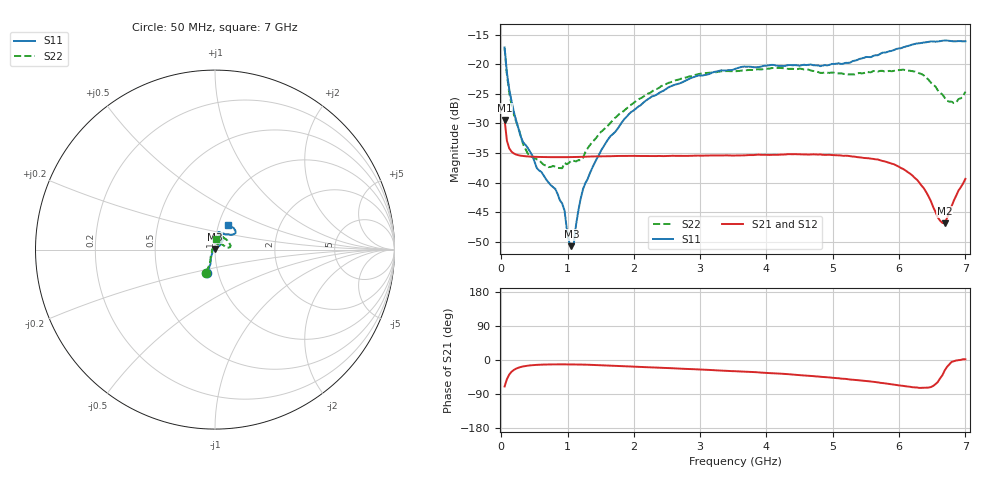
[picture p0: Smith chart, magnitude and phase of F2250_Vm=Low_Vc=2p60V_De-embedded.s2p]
! Integrated Device Technology
! Corporate Headquarters
! 6024 Silver Creek Valley Road
! San Jose, CA 95138  USA
! Phone:  1-408-284-8200
! Toll Free:  1-800-223-1366
! Webpage:  http://www.idt.com/
! Timing and RF Division
! 515 Groton Road, Suite 102
! Westford, MA 01886-6024
! Device:  F2250
! Description: Voltage Variable RF Attenuator
! Frequency:  50.0 -  6000.00 MHz
! Package:  3x3 mm Thin QFN Plastic Package: 16 pin
! Ports:  2 RF, 3 DC
!  Pin  1  = GND
!  Pin  2  = NC
!  Pin  3  = RF1  = Port 1
!  Pin  4  = NC
!  Pin  5  = GND
!  Pin  6  = GND
!  Pin  7  = GND
!  Pin  8  = GND
!  Pin  9  = NC
!  Pin 10  = RF2  = Port 2
!  Pin 11  = NC
!  Pin 12  = GND
!  Pin 13  = GND
!  Pin 14  = VCNTRL
!  Pin 15  = VDD
!  Pin 16  = VMODE
! Vcntrl:  2.600 Volts
! Vmode:  +0.000 Volts
! Vdd:  +3.30  Volts
! Current:  1.176 mA
! Data:  The device was measured on a the F2250 evaluation board which has
!  individual transmission lines to the RF pins.  Data was collected
!  using a calibrated network analyzer.  The evaluation board was
!  de-embedded using a TRL calibration technique.
!  The reference plane is the edge of the package pin.
! Misc:  SN 10
!  Action Tracker AT0258
! Date Measured:  2014-11-26
! Date:  2015-10-15  MJV
! Note:
!  Integrated Device Technology supplies this data as a sample of measured
!  data at the package pin for this product.  Your particular data for this
!  product may vary.
!  Data was taken at 25 degrees C.
!  Integrated Device Technology reserves the right to change this data at anytime.
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# GHz S dB R 50
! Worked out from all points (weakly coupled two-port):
!   201 points, 50 MHz to 7 GHz, reference 50 ohm
!   highest |S21| = -29.41 dB at 50 MHz (marker M1); lowest = -46.8 dB at 6.687 GHz (marker M2)
!   lowest |S11| = -50.7 dB at 1.058 GHz (marker M3), VSWR 1.01, Z = 49.8 + j0.243 ohm
!   |S11| at or under -10 dB: start of sweep to end of sweep
!   |S22| runs from -37.5 to -17.3 dB; largest |S21 - S12| = 6.2e-05
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0.05  -17.18 -108.6  -29.41 -69.8  -29.41 -69.8  -17.28 -111.0
0.08475  -21.45 -107.5  -32.92 -50.4  -32.92 -50.4  -21.74 -110.2
0.15425  -26.23 -116.6  -34.76 -31.1  -34.75 -31.2  -26.81 -122.5
0.29325  -32.21 -127.8  -35.43 -18.5  -35.43 -18.5  -32.09 -137.4
0.3975  -34.09 -141.7  -35.56 -15.0  -35.56 -15.0  -35.05 -160.5
0.91875  -43.51 157.9  -35.69 -11.5  -35.69 -11.5  -37.54 133.5
0.9535  -44.66 170.2  -35.68 -11.5  -35.68 -11.5  -36.65 131.0
1.023  -49.98 143.9  -35.67 -11.6  -35.67 -11.6  -36.63 115.9
1.05775  -50.70 123.4  -35.67 -11.6  -35.67 -11.6  -36.26 110.6
1.0925  -50.41 89.4  -35.66 -11.7  -35.66 -11.7  -36.30 106.4
1.162  -44.71 57.0  -35.64 -11.9  -35.64 -11.9  -36.19 95.5
1.2315  -41.11 44.2  -35.61 -12.1  -35.61 -12.1  -35.80 85.6
1.6485  -32.11 41.9  -35.52 -14.6  -35.52 -14.7  -29.87 64.5
1.96125  -28.04 42.1  -35.46 -17.2  -35.46 -17.2  -26.82 56.8
2.37825  -24.87 47.3  -35.48 -20.3  -35.48 -20.3  -23.99 56.8
3.525  -20.80 72.5  -35.40 -29.5  -35.41 -29.5  -21.19 74.7
4.7065  -20.17 72.3  -35.20 -42.5  -35.20 -42.6  -21.14 72.3
5.85325  -17.81 40.5  -36.64 -63.3  -36.64 -63.3  -21.13 23.0
6.27025  -16.50 40.0  -39.49 -72.6  -39.50 -72.6  -21.36 9.7
6.68725  -15.99 48.8  -46.84 -27.8  -46.82 -27.3  -25.65 28.5
6.861  -16.13 55.1  -42.18 -1.3  -42.13 -1.3  -26.46 57.9
7  -16.13 63.2  -39.34 1.9  -39.30 1.7  -24.62 83.2
